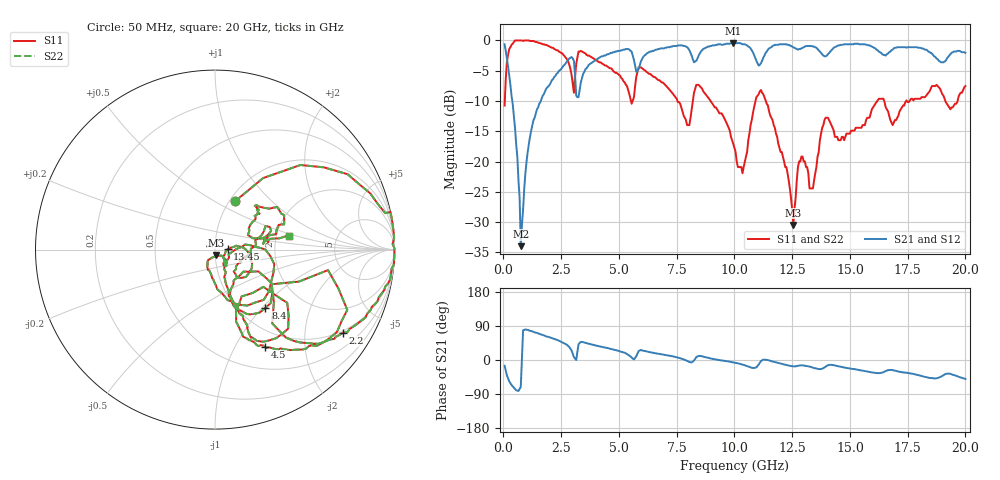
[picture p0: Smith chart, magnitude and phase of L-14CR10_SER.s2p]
#	mhz	s	ma	r	50
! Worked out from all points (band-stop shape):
!   400 points, 50 MHz to 20 GHz, reference 50 ohm
!   highest |S21| = -0.45 dB at 9.95 GHz (marker M1); lowest = -34.0 dB at 750 MHz (marker M2)
!   |S21| within 3 dB of the highest: 8.313 GHz to 10.96 GHz (2.649 GHz wide, 27.5 % of centre); 11.19 GHz to 18.89 GHz (7.699 GHz wide, 51.2 % of centre)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
!   lowest |S11| = -30.5 dB at 12.55 GHz (marker M3), VSWR 1.06, Z = 50.5 - j2.97 ohm
!   |S11| at or under -10 dB: 8.969 GHz to 10.91 GHz (1.942 GHz wide, 19.5 % of centre); 11.36 GHz to 16.18 GHz (4.822 GHz wide, 35 % of centre); 16.48 GHz to 17.43 GHz (947.2 MHz wide, 5.59 % of centre)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
!   |S22| runs from -30.5 to 0.0 dB; largest |S21 - S12| = 0
!   S11 on the Smith chart (normalised r, x): 50 MHz: 1.06, +0.62; 2.2 GHz: 0.93, -3.11; 4.5 GHz: 0.77, -1.33; 8.4 GHz: 1.31, -1.05; 13.45 GHz: 1.15, +0.00; 20 GHz: 2.35, +0.44
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50  0.29 67.6  0.93 -15.3  0.93 -15.3  0.29 67.6
600  1 10.1  0.11 -80.7  0.11 -80.7  1 10.1
750  1 5.6  0.02 -71.0  0.02 -71.0  1 5.6
1200  0.99 -7.1  0.18 76.3  0.18 76.3  0.99 -7.1
2200  0.85 -33.1  0.5 55.5  0.5 55.5  0.85 -33.1
3000  0.44 -41.8  0.71 16.4  0.71 16.4  0.44 -41.8
3150  0.64 -10.3  0.35 0.0  0.35 0.0  0.64 -10.3
3400  0.81 -36.7  0.49 47.6  0.49 47.6  0.81 -36.7
4500  0.61 -62.7  0.77 31.6  0.77 31.6  0.61 -62.7
6700  0.47 -67.5  0.85 16.4  0.85 16.4  0.47 -67.5
7950  0.2 -58.6  0.88 -2.2  0.88 -2.2  0.2 -58.6
8400  0.43 -49.2  0.71 9.3  0.71 9.3  0.43 -49.2
9950  0.14 -64.4  0.95 -6.2  0.95 -6.2  0.14 -64.4
10050  0.12 -64.9  0.95 -7.5  0.95 -7.5  0.12 -64.9
11150  0.39 -45.9  0.65 -2.7  0.65 -2.7  0.39 -45.9
12550  0.03 -77.9  0.88 -16.8  0.88 -16.8  0.03 -77.9
12900  0.11 -54.5  0.86 -14.2  0.86 -14.2  0.11 -54.5
13350  0.06 -27.0  0.9 -19.3  0.9 -19.3  0.06 -27.0
13450  0.07 1.2  0.89 -21.1  0.89 -21.1  0.07 1.2
13950  0.23 -27.2  0.74 -17.3  0.74 -17.3  0.23 -27.2
16700  0.24 15.2  0.8 -26.5  0.8 -26.5  0.24 15.2
20000  0.42 10.5  0.79 -50.0  0.79 -50.0  0.42 10.5
